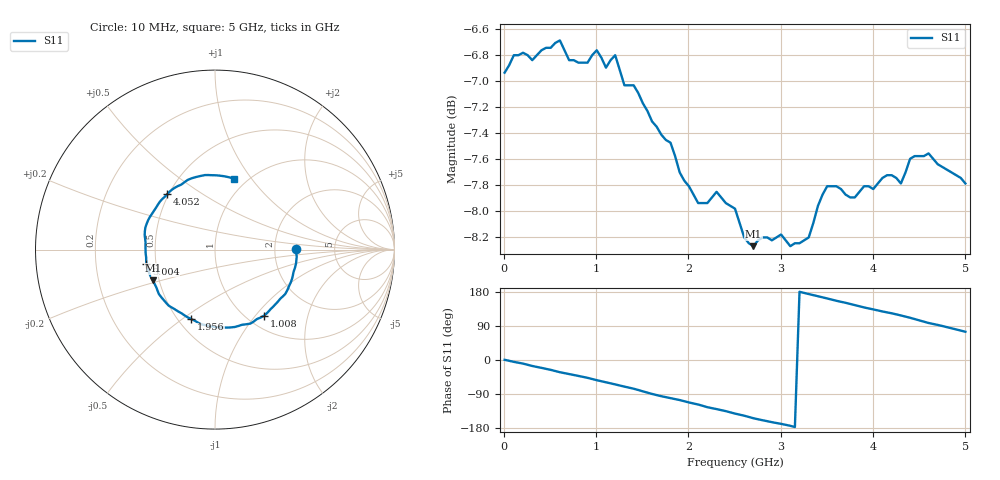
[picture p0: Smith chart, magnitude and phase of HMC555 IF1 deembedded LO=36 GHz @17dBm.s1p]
!Hittite Microwave Corporation
!20 Alpha Road
!Chelmsford, MA 01824
!Tel: 978-250-3343
!Fax: 978-250-3373
!Device: HMC555, 32-38GHz, I/Q Mixer
!Misc: IF1 Return Loss with LO = 36 GHz @ 17 dBm, Data includes one K connector, Room
# MHZ S MA R 50
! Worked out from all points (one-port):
!   101 points, 10 MHz to 5 GHz, reference 50 ohm
!   lowest |S11| = -8.3 dB at 2.705 GHz (marker M1), VSWR 2.26, Z = 23.1 - j9.29 ohm
!   |S11| at or under -10 dB: nowhere
!   S11 on the Smith chart (normalised r, x): 10 MHz: 2.64, +0.03; 1.008 GHz: 1.19, -1.11; 1.956 GHz: 0.58, -0.54; 3.004 GHz: 0.44, -0.08; 4.052 GHz: 0.49, +0.36; 5 GHz: 0.88, +0.83
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10  0.45 0.5
209.6  0.458 -9.5
459.1  0.46 -23.4
658.7  0.459 -34.7
1008  0.459 -53.3
1257.5  0.451 -67.3
1407.2  0.445 -75.7
1556.9  0.435 -86.2
1706.6  0.426 -95.5
1906.2  0.412 -105.7
1956.1  0.409 -108.8
2205.6  0.401 -124.5
2305.4  0.405 -129.6
2505  0.399 -141.4
2704.6  0.386 -153.7
3004  0.39 -168.5
3153.7  0.387 -176.8
3303.4  0.389 174.1
3503  0.407 162.4
3752.5  0.403 147.9
3902.2  0.407 138.8
4051.9  0.408 130.8
4201.6  0.411 123.3
4301.4  0.408 117.5
4401.2  0.417 111.4
4600.8  0.419 97.7
4800.4  0.413 86.7
5000  0.408 74.6
